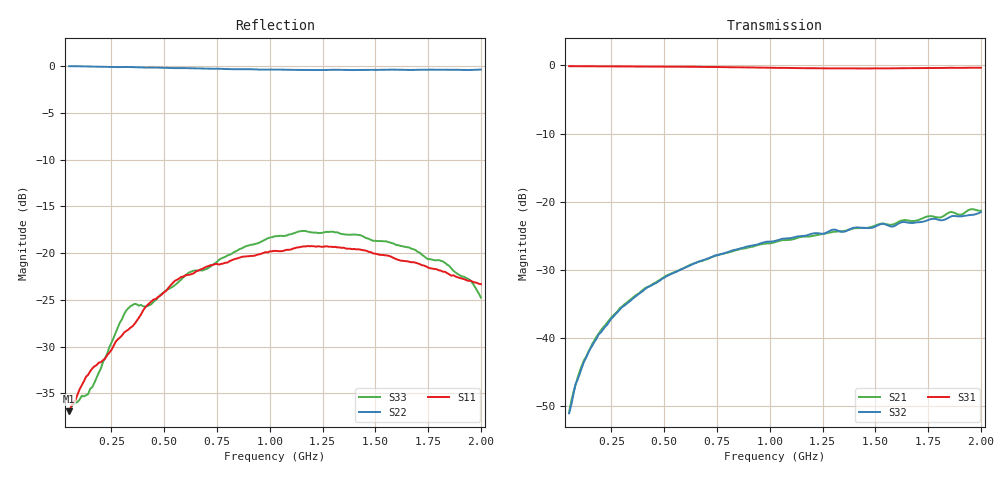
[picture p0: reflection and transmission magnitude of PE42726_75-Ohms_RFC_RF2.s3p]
! Created Wed Feb  7 16:17:06 2024
# hz S db R 75
! 3 Port Network Data from Sweep2.SP1.SP block
! freq  dbS11  angS11  dbS12  angS12  dbS13  angS13
!  dbS21  angS21
!  dbS22  angS22  dbS23  angS23
!  dbS31  angS31  dbS32  angS32
!  dbS33  angS33
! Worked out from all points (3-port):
!   196 points, 50 MHz to 2 GHz, reference 75 ohm
!   strongest paths, dB at 50 MHz, 540 MHz, 1.03 GHz, 1.52 GHz, 2 GHz:
!     S31: -0.1, -0.2, -0.4, -0.4, -0.3
!     S32: -51.1, -30.5, -25.7, -23.4, -21.5
!     S21: -50.9, -30.5, -25.9, -23.3, -21.3
!   lowest |S11| = -36.9 dB at 50 MHz (marker M1), VSWR 1.03, Z = 76.9 - j1.02 ohm
!   |S11| at or under -10 dB: start of sweep to end of sweep
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5e7  -36.90 -27.6  -50.35 85.4  -0.11 -0.9
     -50.91 87.1  -0.01 -8.0  -50.39 83.9
     -0.11 -0.9  -51.07 83.0  -37.12 -33.1
1.9e8  -31.71 -51.1  -39.37 84.7  -0.12 -3.3
       -39.37 84.5  -0.06 -30.0  -39.41 77.6
       -0.12 -3.2  -39.47 77.2  -32.79 -97.6
3.2e8  -28.32 -67.6  -34.84 80.2  -0.14 -5.5
       -34.90 79.7  -0.10 -50.8  -35.09 69.4
       -0.13 -5.5  -35.05 69.3  -26.15 -122.1
5.4e8  -23.21 -75.7  -30.47 73.6  -0.18 -9.2
       -30.46 73.0  -0.21 -85.4  -30.52 55.0
       -0.18 -9.2  -30.52 55.5  -23.60 -155.4
7.6e8  -21.22 -72.5  -27.80 67.3  -0.25 -12.8
       -27.82 66.7  -0.29 -119.8  -27.79 40.8
       -0.24 -12.9  -27.77 41.6  -20.71 171.2
1.03e9  -19.76 -77.2  -25.78 60.5  -0.35 -16.9
        -25.90 60.9  -0.37 -161.1  -25.88 25.3
        -0.36 -17.0  -25.73 24.7  -18.18 138.4
1.29e9  -19.31 -77.8  -24.41 55.5  -0.40 -20.6
        -24.51 57.1  -0.40 161.2  -24.28 12.4
        -0.44 -20.6  -24.19 10.9  -17.70 109.5
1.56e9  -20.27 -74.4  -23.45 52.6  -0.44 -24.1
        -23.36 53.1  -0.38 124.8  -23.40 -2.3
        -0.43 -24.2  -23.50 -3.0  -18.80 77.4
1.77e9  -21.65 -65.9  -22.59 51.8  -0.37 -27.3
        -22.15 51.5  -0.38 98.0  -22.01 -9.9
        -0.39 -27.5  -22.52 -9.6  -20.69 50.9
2e9  -23.31 -37.9  -21.55 51.9  -0.32 -31.0
     -21.34 50.7  -0.37 69.4  -21.28 -18.4
     -0.34 -30.9  -21.53 -17.1  -24.75 21.0
